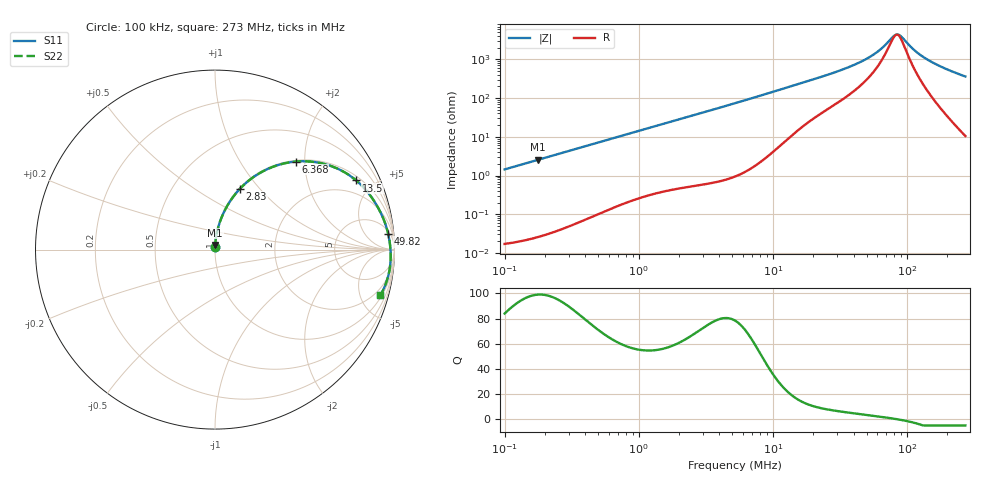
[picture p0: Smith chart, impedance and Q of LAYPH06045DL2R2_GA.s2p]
! LAYPH06045DL2R2_GA  S-PARAMETER MODEL  ( General Type )
! Model Generated by TAIYO YUDEN Corporation (http://www.ty-top.com)
! Version 2.0
! TAIYO YUDEN Control No. 180914NI43SB-FBB
! Copyright(c) 2018 TAIYO YUDEN CO.,LTD. All Rights Reserved.
! Product Description (link to TY-COMPAS)
! https://ds.yuden.co.jp/TYCOMPAS/or/detail?pn=LAYPH06045DL2R2NGA&u=M
! Products Name : Inductors
! Characteristics :
!  Inductance : 2.2 uH , SRF(min) : -Hz , DC Resistance(max) : 0.0169 Ohm
!  Rated Current : Saturation :4.2 A , Temp Rise : 2.8 A (25 degC)
!  Case Size : 6.3 x 6.0 / 0.248 x 0.236 [mm/inch] , Thickness : 4.5 / 0.177 [mm/inch]
!  (Conditions: Temperature = 25 degC , DC Bias Current/Voltage = 0A / 0V)
! External Node Assignments :
!  1  o---GGG---o  2
! GND o---------o GND
! Frequency Range : 0.1MHz  -  272.98108MHz  [ 402 STEP ]
# MHz S RI R 50
! Freq[MHz].  S11 Real  S11 Imag  S21 Real  S21 Imag  S12 Real  S12 Imag  S22 Real  S22 Imag
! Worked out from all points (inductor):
!   401 points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, 100 kHz to 273 MHz, reference 50 ohm
!   read as one part in series: L = 2.28 uH near 104 kHz
!   highest Q = 98.9 at 177.5 kHz (marker M1), where L = 2.28 uH
!   self-resonance near 84 MHz
!   S11 on the Smith chart (normalised r, x): 100 kHz: 1.00, +0.03; 2.83 MHz: 1.01, +0.79; 6.368 MHz: 1.03, +1.80; 13.5 MHz: 1.20, +3.97; 49.82 MHz: 7, +20; 273 MHz: 1.21, -7.20
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0.1  0.000377 0.0143  0.9996 -0.0143  0.9996 -0.0143  0.000377 0.0143
0.177468  0.000905 0.0254  0.9991 -0.0254  0.9991 -0.0254  0.000905 0.0254
0.376316  0.00355 0.0536  0.9965 -0.0536  0.9965 -0.0536  0.00355 0.0536
0.767015  0.0135 0.1074  0.9865 -0.1074  0.9865 -0.1074  0.0135 0.1074
1.416134  0.0415 0.1906  0.9585 -0.1906  0.9585 -0.1906  0.0415 0.1906
2.829867  0.1392 0.3392  0.8608 -0.3392  0.8608 -0.3392  0.1392 0.3392
5.329134  0.3621 0.4742  0.6379 -0.4742  0.6379 -0.4742  0.3621 0.4742
6.367509  0.4488 0.4902  0.5512 -0.4902  0.5512 -0.4902  0.4488 0.4902
8.912617  0.618 0.4747  0.382 -0.4747  0.382 -0.4747  0.618 0.4747
13.50213  0.7867 0.3853  0.2133 -0.3853  0.2133 -0.3853  0.7867 0.3853
19.66158  0.877 0.2845  0.123 -0.2845  0.123 -0.2845  0.877 0.2845
34.20958  0.9436 0.1585  0.0564 -0.1585  0.0564 -0.1585  0.9436 0.1585
49.81545  0.9648 0.0879  0.0352 -0.0879  0.0352 -0.0879  0.9648 0.0879
61.92381  0.9719 0.0507  0.0281 -0.0507  0.0281 -0.0507  0.9719 0.0507
73.9896  0.9758 0.0211  0.0242 -0.0211  0.0242 -0.0211  0.9758 0.0211
81.68124  0.9773 0.00469  0.0227 -0.00469  0.0227 -0.00469  0.9773 0.00469
86.6749  0.978 -0.00527  0.022 0.00527  0.022 0.00527  0.978 -0.00527
91.97384  0.9785 -0.0153  0.0215 0.0153  0.0215 0.0153  0.9785 -0.0153
114.3294  0.9785 -0.0539  0.0215 0.0539  0.0215 0.0539  0.9785 -0.0539
139.3353  0.9755 -0.092  0.0245 0.092  0.0245 0.092  0.9755 -0.092
191.2082  0.9611 -0.1617  0.0389 0.1617  0.0389 0.1617  0.9611 -0.1617
272.9811  0.9221 -0.254  0.0779 0.254  0.0779 0.254  0.9221 -0.254
